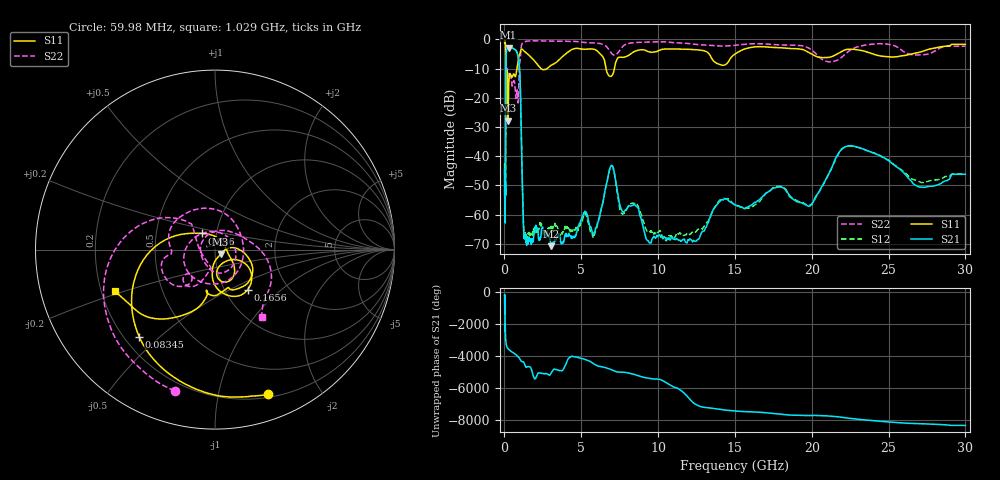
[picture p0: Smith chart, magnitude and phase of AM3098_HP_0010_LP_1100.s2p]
! Date/Time: Thu, Feb 28, 2019 8:33 AM
! Network Analyzer: Agilent Technologies E8364B Rev: A.07.50.67
! Sweep from 0.010 to 30.000 GHz, 1601 Points, Sweep Type: LOG
! Power Supply: 5.023 V, 0.002 A
# Hz S DB R 50
!freq MagS11 AngS11 MagS21 AngS21 MagS12 AngS12 MagS22 AngS22
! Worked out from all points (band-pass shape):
!   1601 points, 10 MHz to 30 GHz, reference 50 ohm
!   highest |S21| = -2.79 dB at 267.8 MHz (marker M1); lowest = -70.8 dB at 3.032 GHz (marker M2)
!   |S21| within 3 dB of the highest: 107.1 MHz to 888.2 MHz (781 MHz wide, 157 % of centre)
!   lowest |S11| = -27.9 dB at 233.9 MHz (marker M3), VSWR 1.08, Z = 53.1 - j2.79 ohm
!   |S11| at or under -10 dB: 92.11 MHz to 811.4 MHz (719.3 MHz wide, 159 % of centre); 2.375 GHz to 2.772 GHz (397.2 MHz wide, 15.4 % of centre); 6.613 GHz to 7.156 GHz (542.3 MHz wide, 7.88 % of centre)
!   |S22| runs from -22.5 to -0.5 dB; largest |S21 - S12| = 0.012
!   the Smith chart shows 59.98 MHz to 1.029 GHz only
!   S11 on the Smith chart (normalised r, x): 59.98 MHz: 0.23, -1.41; 83.45 MHz: 0.26, -0.43; 96 MHz: 0.85, +0.16; 165.6 MHz: 1.27, -0.62; 1.029 GHz: 0.26, -0.19
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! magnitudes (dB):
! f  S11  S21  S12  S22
! 10 MHz  -0.4  -44.4  -43.1  -0.6
! 38.04 MHz  -0.5  -61.8  -59.2  -1.0
! 59.98 MHz  -1.3  -50.8  -51.7  -1.7
! 83.45 MHz  -3.8  -33.9  -33.6  -4.3
! 96 MHz  -18.8  -11.1  -11.0  -21.3
! 144.7 MHz  -15.1  -3.5  -3.4  -12.9
! 165.6 MHz  -10.8  -3.4  -3.3  -10.2
! 233.9 MHz  -27.9  -2.9  -2.8  -12.1
! 267.8 MHz  -17.0  -2.8  -2.8  -12.3
! 550.5 MHz  -12.3  -3.1  -3.0  -14.9
! 885.5 MHz  -7.7  -5.7  -5.7  -21.7
! 1.029 GHz  -4.4  -15.7  -15.7  -6.8
! 1.27 GHz  -4.0  -67.7  -66.2  -0.9
! 2.084 GHz  -8.2  -64.3  -66.3  -0.5
! 3.032 GHz  -8.9  -70.8  -64.0  -0.6
! 5.812 GHz  -3.3  -66.3  -67.5  -1.2
! 6.924 GHz  -12.6  -43.3  -43.4  -4.4
! 7.926 GHz  -5.9  -58.4  -58.6  -1.6
! 12.19 GHz  -3.5  -68.8  -66.1  -1.5
! 19.8 GHz  -4.5  -57.2  -56.8  -3.0
! 22.56 GHz  -3.4  -36.3  -36.5  -3.5
! 30 GHz  -1.7  -46.2  -46.1  -2.3
